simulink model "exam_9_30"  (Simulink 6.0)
settings: Solver=ode45  StartTime=0.0  StopTime=10.0  RelTol=1e-3

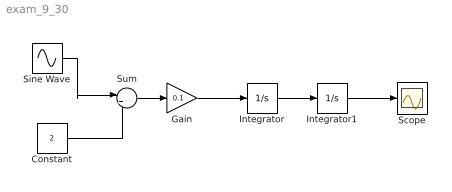
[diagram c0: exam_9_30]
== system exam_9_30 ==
  Constant : Constant  Value=2
  Gain : Gain  Gain=0.1
  Integrator : Integrator
  Integrator1 : Integrator
  Scope : Scope
  Sine Wave : Sin  SampleTime=0
  Sum : Sum  Inputs=|++
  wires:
  Sine Wave/1 -> Sum/1
  Constant/1 -> Sum/2
  Sum/1 -> Gain/1
  Gain/1 -> Integrator/1
  Integrator/1 -> Integrator1/1
  Integrator1/1 -> Scope/1
